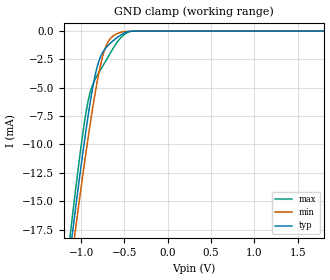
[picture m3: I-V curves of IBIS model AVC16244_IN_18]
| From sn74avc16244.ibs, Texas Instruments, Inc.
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[Model]   AVC16244_IN_18
Model_type  Input
Vinl=0.5775
Vinh=1.2675
| variable   typ   min   max
C_comp   4.13pF   3.12pF   5.77pF
[Temperature Range]   40   100   -40
| Ambient temperature   25   85   -40
[Voltage range]   1.8   1.65   1.95
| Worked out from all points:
|   GND clamp passes 1 mA (typ) near -0.65 V on its own axis
[GND Clamp]
| AVC16244_IN_18
|   Voltage   I(typ)   I(min)   I(max)
-1.8V     -63.94mA   -63.47mA   -65.85mA
-1.125V   -19.34mA   -21mA      -17.92mA
-1.095V   -17.49mA   -19.23mA   -15.96mA
-1.065V   -15.67mA   -17.48mA   -14.04mA
-935mV    -8.266mA   -10.23mA   -6.794mA
-890mV    -6.034mA   -7.912mA   -5.246mA
-830mV    -3.615mA   -5.101mA   -4.13mA
-780mV    -2.328mA   -3.134mA   -3.457mA
-725mV    -1.582mA   -1.574mA   -2.749mA
-615mV    -754.2uA   -343.5uA   -1.327mA
-420mV    -16.52uA   -11.44uA   -21.14uA
1.8V      203pA      695.1pA    11.5pA
